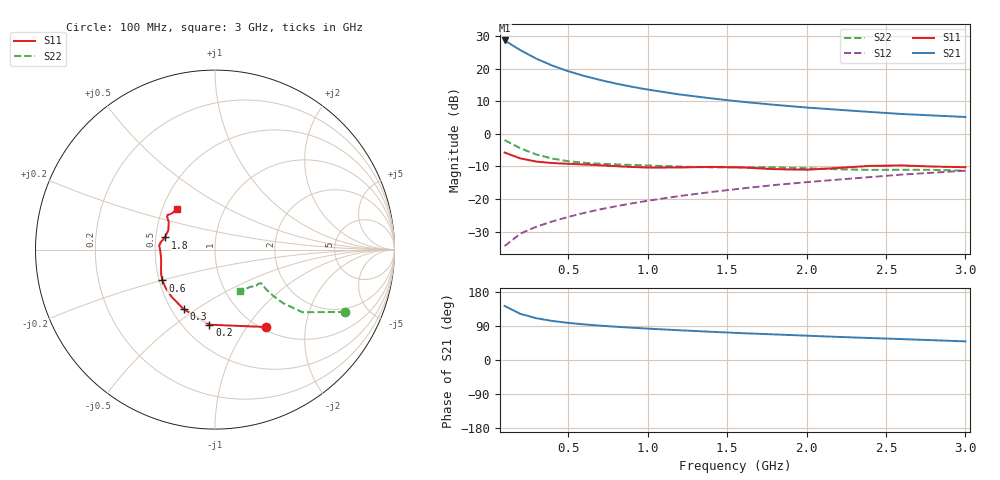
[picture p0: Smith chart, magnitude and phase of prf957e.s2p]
! Filename:  PRF957E.S2P  Version:  3.0
! Philips part #:  PRF957  Date:  Nov 1998
! Bias condition:  Vce=3V, Ic=15mA
#  MHz  S  MA  R 50
! Freq  S11  S21  S12  S22
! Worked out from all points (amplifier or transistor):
!   20 points, 100 MHz to 3 GHz, reference 50 ohm
!   highest |S21| = 28.7 dB at 100 MHz (marker M1)
!   |S21| within 3 dB of that: start of sweep to 200.1 MHz
!   unconditionally stable (mu >= 1): 863.3 MHz to end of sweep
!   at 400 MHz: K = 0.82, MSG = 23.9 dB, |S12| = -26.9 dB
!   at 1.2 GHz: K = 1.04, MAG = 14.4 dB, |S12| = -19.1 dB
!   at 3 GHz: K = 1.04, MAG = 7.1 dB, |S12| = -11.3 dB
!   S11 on the Smith chart (normalised r, x): 100 MHz: 1.05, -1.24; 200 MHz: 0.67, -0.68; 300 MHz: 0.58, -0.45; 600 MHz: 0.52, -0.20; 1.8 GHz: 0.56, +0.08; 3 GHz: 0.60, +0.30
100  0.517 -56.6  27.12 142.5  0.01893 69.2  0.8044 -25.6
200  0.4195 -94.2  19.2 121.7  0.0296 63.6  0.5991 -35.6
300  0.3753 -117.7  14.24 110.2  0.03768 63.9  0.4824 -38.2
400  0.3571 -132.7  11.17 103.0  0.04535 65.8  0.4177 -38.5
500  0.3475 -142.6  9.16 97.9  0.05319 67.7  0.3813 -38.2
600  0.3396 -149.6  7.755 94.0  0.06118 69.3  0.3604 -37.8
700  0.3302 -155.1  6.718 90.7  0.06933 70.5  0.3483 -37.4
800  0.3199 -160.1  5.924 87.8  0.07747 71.6  0.3405 -36.8
900  0.3107 -165.1  5.29 85.2  0.0857 72.5  0.3338 -36.3
1000  0.3047 -170.1  4.786 82.8  0.09414 73.0  0.3275 -36.0
1200  0.3053 -178.8  4.03 78.5  0.1112 73.7  0.3148 -36.5
1400  0.3118 175.8  3.508 74.4  0.1283 73.9  0.3068 -38.7
1600  0.305 172.2  3.101 70.7  0.1459 73.9  0.306 -41.0
1800  0.2875 166.4  2.788 67.5  0.1642 73.6  0.3052 -42.4
2000  0.2817 157.2  2.539 64.2  0.1816 73.3  0.2977 -43.6
2200  0.3002 149.2  2.345 60.9  0.1989 72.9  0.286 -46.4
2400  0.3227 145.6  2.17 58.0  0.2173 72.1  0.28 -50.5
2600  0.3278 144.1  2.019 55.2  0.2375 71.2  0.2813 -54.2
2800  0.3151 140.7  1.914 52.2  0.2541 70.7  0.2804 -56.4
3000  0.3081 133.4  1.817 49.2  0.2723 70.2  0.2718 -58.7
